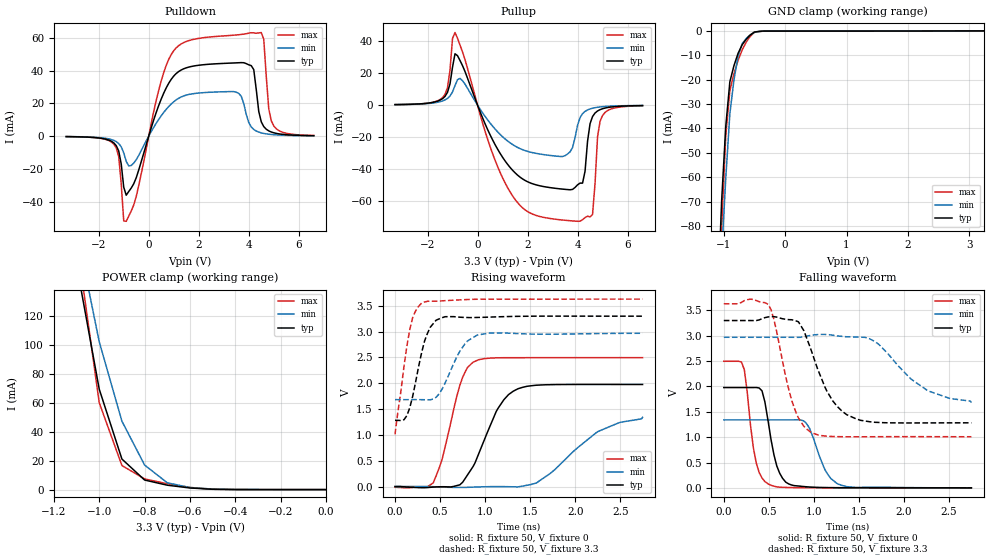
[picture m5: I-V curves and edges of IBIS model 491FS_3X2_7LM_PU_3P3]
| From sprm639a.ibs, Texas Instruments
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|BQ0491FS_3X2_7LM_PZ_3P3; PULLUP_OFF
|   Model Cell 491FS_3X2_7LM_PU_3P3
|BQ0491FS_3X2_7LM_PU_3P3
[Model]   491FS_3X2_7LM_PU_3P3
Model_type   I/O
Polarity   Non-Inverting
Enable   Active-Low
Vinl =  1.25
Vinh =  1.65
Cref =  15.0001pF
Rref =  101.0000M
Vref =  0V
Vmeas =  1.65
C_comp   1.2p   1.2p   1.2p
[Model Spec]
Vinl   1.25   1.12   1.38
Vinh   1.65   1.45   1.75
[Temperature Range]   25   155   -40
[Voltage Range]   3.3   2.97   3.63
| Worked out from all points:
|   slope of the pulldown table from 0 to 0.495 V, typ, clamps not added: 22 ohm
|   slope of the pullup table from 0 to 0.495 V, typ, clamps not added: 26.9 ohm
|   GND clamp passes 1 mA (typ) near -0.53 V on its own axis
|   POWER clamp passes 1 mA (typ) near -0.59 V on its own axis
|   rising waveform, R_fixture 50, V_fixture 0: 20-80 % time 300ps typ, 528ps min, 211ps max; typ from 0.001 V to 1.98 V
|   rising waveform, R_fixture 50, V_fixture 3.3: 20-80 % time 158ps typ, 218ps min, 133ps max; typ from 1.28 V to 3.3 V
|   falling waveform, R_fixture 50, V_fixture 0: 20-80 % time 130ps typ, 180ps min, 107ps max; typ from 1.98 V to 0.001 V
|   falling waveform, R_fixture 50, V_fixture 3.3: 20-80 % time 290ps typ, 459ps min, 208ps max; typ from 3.3 V to 1.28 V
[POWER_clamp]
|   voltage   I(typ)   I(min)   I(max)
-3.3V     2.375A     2.63A      3.153A
-1.1V     156mA      180.2mA    173.4mA
-1.067V   127.2mA    154.3mA    135.7mA
-1.033V   98.45mA    128.4mA    97.99mA
-1V       69.65mA    102.5mA    60.28mA
-900mV    21.19mA    47.43mA    16.7mA
-800mV    6.636mA    17.03mA    7.395mA
-700mV    3.052mA    4.718mA    4.065mA
-600mV    1.132mA    1.432mA    1.49mA
-500mV    224.9uA    381.2uA    256.9uA
0V        310pA      5.943nA    270.6pA
[Pulldown]
|   voltage   I(typ)   I(min)   I(max)
-3.3V     -269.8uA   -248.1uA   -260.2uA
-1.4V     -4.056mA   -2.548mA   -4.78mA
-1.2V     -9.105mA   -4.482mA   -12.53mA
-900mV    -36.12mA   -15.43mA   -52.09mA
1V        36.78mA    21.07mA    52.28mA
3.5V      44.86mA    26.92mA    61.93mA
4.1V      43.14mA    5.644mA    63.29mA
4.5V      8.805mA    2.025mA    63.4mA
4.6V      5.861mA    1.678mA    59.29mA
4.8V      3.241mA    1.203mA    16.69mA
5V        2.072mA    900.6uA    6.272mA
6.6V      302.2uA    232.4uA    414.2uA
[Pullup]
|   voltage   I(typ)   I(min)   I(max)
-3.3V     296.7uA    284.3uA    270.4uA
-1.4V     3.997mA    2.582mA    4.655mA
-1.2V     8.017mA    4.201mA    10.97mA
-900mV    32.15mA    12.24mA    45.44mA
1.4V      -40.82mA   -24.72mA   -56.86mA
3.4V      -52.65mA   -32.22mA   -72.03mA
4V        -49.98mA   -12.64mA   -72.82mA
4.2V      -48.91mA   -5.386mA   -71.83mA
4.6V      -7.16mA    -1.965mA   -68.53mA
4.8V      -3.684mA   -1.373mA   -19.8mA
5V        -2.282mA   -1.01mA    -6.487mA
6.6V      -316.6uA   -254.8uA   -401.1uA
[GND_clamp]
|   voltage   I(typ)   I(min)   I(max)
-3.3V     -1.947A    -1.623A    -3.254A
-1.1V     -112mA     -127.1mA   -135.8mA
-1.033V   -69.63mA   -91.64mA   -80.2mA
-966.7mV  -39.25mA   -60.63mA   -43.14mA
-900mV    -20.89mA   -34.03mA   -24.56mA
-833.3mV  -14.31mA   -20.14mA   -17.7mA
-766.7mV  -9.259mA   -10.54mA   -12.12mA
-700mV    -5.75mA    -5.239mA   -7.84mA
-566.7mV  -1.652mA   -1.618mA   -2.192mA
-500mV    -488.4uA   -632.2uA   -598.3uA
-300mV    -87.1uA    -54.14uA   -139.1uA
3.233V    -4.592uA   15.73uA    -37.4uA
[Ramp]
| variable   typ   min   max
dV/dt_f   1.259329/0.2952073n   0.811572/0.4795714n   1.628978/0.2136225n
dV/dt_r   1.201068/0.3057452n  0.8158006/0.5348986n   1.513193/0.2081101n
R_load = 50
[Rising Waveform]
R_fixture = 50
V_fixture = 0
V_fixture_min = 0
V_fixture_max = 0
|   time   V(typ)   V(min)   V(max)
0s        1.151mV    970.9uV    -13.17mV
424ps     -9.867mV   -2.288mV   70.84mV
524ps     -2.864mV   -10.93mV   533.9mV
720ps     33.88mV    -16.4mV    1.964V
868ps     392mV      -10.45mV   2.41V
1.124ns   1.456V     -662.8uV   2.492V
1.364ns   1.894V     -6.363mV   2.496V
1.72ns    1.973V     250.2mV    2.497V
2.26ns    1.978V     1.072V     2.497V
2.748ns   1.977V     1.34V      2.497V
[Rising Waveform]
R_fixture = 50
V_fixture = 3.3
V_fixture_min = 2.97
V_fixture_max = 3.63
|   time   V(typ)   V(min)   V(max)
0s        1.284V     1.684V     1.012V
100ps     1.295V     1.684V     2.332V
164ps     1.528V     1.684V     3.04V
228ps     2.017V     1.684V     3.399V
296ps     2.597V     1.683V     3.553V
360ps     2.967V     1.679V     3.588V
456ps     3.221V     1.73V      3.59V
720ps     3.28V      2.621V     3.615V
912ps     3.275V     2.933V     3.628V
2.748ns   3.3V       2.969V     3.63V
[Falling Waveform]
R_fixture = 50
V_fixture = 0
V_fixture_min = 0
V_fixture_max = 0
|   time   V(typ)   V(min)   V(max)
0s        1.979V     1.341V     2.497V
228ps     1.979V     1.341V     2.33V
360ps     1.98V      1.341V     494.2mV
424ps     1.915V     1.341V     197.5mV
492ps     1.317V     1.341V     79.65mV
588ps     434mV      1.341V     21.59mV
752ps     57.65mV    1.341V     6.972mV
932ps     20.63mV    1.232V     3.778mV
1.26ns    4.696mV    82.83mV    1.871mV
2.748ns   1.286mV    1.497mV    1.361mV
[Falling Waveform]
R_fixture = 50
V_fixture = 3.3
V_fixture_min = 2.97
V_fixture_max = 3.63
|   time   V(typ)   V(min)   V(max)
0s        3.3V       2.97V      3.63V
492ps     3.371V     2.97V      3.62V
752ps     3.316V     2.97V      1.735V
828ps     3.276V     2.969V     1.382V
976ps     2.684V     3.01V      1.086V
1.144ns   1.909V     3.024V     1.019V
1.364ns   1.444V     2.979V     1.008V
1.672ns   1.294V     2.89V      1.009V
2.26ns    1.282V     1.921V     1.01V
2.748ns   1.283V     1.683V     1.009V
